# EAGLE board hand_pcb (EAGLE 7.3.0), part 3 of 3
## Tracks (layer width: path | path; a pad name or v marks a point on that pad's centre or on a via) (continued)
N$80 (continued)
  Top 0.381: C64.1 102.23,75.46 102.23,77.09 104.59,79.45 THMB3.9
N$81
  Top 0.381: THMB3.12 107.83,77.36 108.33,76.86 108.33,75.6 C65.1
N$82
  Top 0.381: PKYRNG3.12 105.34,109.19 106.53,110.85 106.81,111.06 107.37,111.91 108.84,111.91 C62.1
N$83
  Top 0.381: C59.1 138.01,108.27 INDMID3.12
N$84
  Top 0.254: O3.3 90.39,81.51 | 92.99,84.48 93.06,84.47 HAND_MICRO3.33
  Top 0.508: 90.39,81.51 91.54,81.51 92.99,82.92 92.99,84.48
N$85
  Top 0.254: O3.1 88.88,83.64 | 91.47,86.31 HAND_MICRO3.32
  Top 0.508: 88.88,83.64 88.88,84.25 90.96,86.31 91.47,86.31
N$86
  Top 0.254: RST3.P$1 85.18,96.05 BOOTLOADER3.10
N$87
  Top 0.254: R51.2 96.36,98.58 95.12,98.58 94.61,98.06 HAND_MICRO3.13
N$88  (via drill 0.38)
  Top 0.254: 94.28,100.87 C68.1 95.43,100.94 95.43,102.31 96.04,102.92 96.72,102.92 97.36,102.28 R51.1 | 94.28,100.87 C67.1 | 94.28,100.87 94.28,98.81 94.11,98.63 HAND_MICRO3.14 94.11,94.92 v93.93,94.59
  Bottom 0.254: v93.93,94.59 94,93.52 U$39.2
N$89  (via drill 0.38)
  Top 0.254: HAND_MICRO3.17 89.62,93.97 v89.59,94 | v91.57,97.89 91.24,97.89 90.47,98.65 90.47,100.38 90.97,100.87 C69.1
  Bottom 0.254: v89.59,94 89.59,95.91 v91.57,97.89
N$90  (via drill 0.38)
  Top 0.254: USB3.4 83.06,105.66 84.23,105.69 84.81,105.11 v84.81,100.53 | v92.59,91.25 92.39,91.25 92.13,90.98 HAND_MICRO3.23 | BOOTLOADER3.6 87.16,90.35 88.19,90.35 v88.72,89.43
  Bottom 0.254: v84.81,100.53 84.81,97.41 90.99,91.25 v92.59,91.25 91.25,89.45 v88.72,89.43
N$91  (via drill 0.38)
  Top 0.254: v109.47,93.45 110.84,93.45 RED3.2
  Bottom 0.254: R62.1 109,92.98 v109.47,93.45
N$92  (via drill 0.38)
  Top 0.254: GREEN3.2 108.96,95.67 v109.98,96.62
  Bottom 0.254: v109.98,96.62 109.79,96.65 R63.1
N$93  (via drill 0.38)
  Top 0.254: v112.62,96.72 111.4,95.83 YELLOW3.2
  Bottom 0.254: R64.1 112.39,96.53 v112.62,96.72
N$94
  Top 0.254: INDMID3.6 128.86,112.05 IMF3.P$1
N$95
  Top 0.254: PKYRNG3.6 102.03,104.73 100.84,103.53 PYF3.P$1
N$96
  Top 0.254: THMB3.6 103.33,82.05 TF3.P$1
OSC
  pour Route15 (isolate 0.406, rank 6): 12.79,13.22 16,13.22 16,13.97 16.9,13.97 18.52,15.58 18.52,17.86 16.87,19.51 15.28,19.51 13.07,17.3 12.79,17.3
  pour Bottom (isolate 0.406, rank 6): 12.79,13.22 16,13.22 16,13.97 16.9,13.97 18.52,15.58 18.52,17.86 16.87,19.51 15.28,19.51 13.07,17.3 12.79,17.3
  pour Route2 (isolate 0.406, rank 6): 12.79,13.22 16,13.22 16,13.97 16.9,13.97 18.52,15.58 18.52,17.86 16.87,19.51 15.28,19.51 13.07,17.3 12.79,17.3
OSC1
  pour Route15 (isolate 0.406, rank 6): 58.97,120.41 55.75,120.41 55.75,119.66 54.85,119.66 53.24,118.05 53.24,115.77 54.89,114.12 56.48,114.12 58.69,116.33 58.97,116.33
  pour Bottom (isolate 0.406, rank 6): 58.97,120.41 55.75,120.41 55.75,119.66 54.85,119.66 53.24,118.05 53.24,115.77 54.89,114.12 56.48,114.12 58.69,116.33 58.97,116.33
  pour Route2 (isolate 0.406, rank 6): 58.97,120.41 55.75,120.41 55.75,119.66 54.85,119.66 53.24,118.05 53.24,115.77 54.89,114.12 56.48,114.12 58.69,116.33 58.97,116.33
OSC2
  pour Route15 (isolate 0.406, rank 6): 133.82,53.25 130.61,53.25 130.61,52.5 129.71,52.5 128.09,50.89 128.09,48.62 129.74,46.96 131.33,46.96 133.54,49.17 133.82,49.17
  pour Bottom (isolate 0.406, rank 6): 133.82,53.25 130.61,53.25 130.61,52.5 129.71,52.5 128.09,50.89 128.09,48.62 129.74,46.96 131.33,46.96 133.54,49.17 133.82,49.17
  pour Route2 (isolate 0.406, rank 6): 133.82,53.25 130.61,53.25 130.61,52.5 129.71,52.5 128.09,50.89 128.09,48.62 129.74,46.96 131.33,46.96 133.54,49.17 133.82,49.17
OSC3
  pour Route15 (isolate 0.406, rank 6): 87.77,80.23 90.98,80.23 90.98,80.98 91.88,80.98 93.5,82.59 93.5,84.86 91.85,86.51 90.26,86.51 88.05,84.3 87.77,84.3
  pour Bottom (isolate 0.406, rank 6): 87.77,80.23 90.98,80.23 90.98,80.98 91.88,80.98 93.5,82.59 93.5,84.86 91.85,86.51 90.26,86.51 88.05,84.3 87.77,84.3
  pour Route2 (isolate 0.406, rank 6): 87.77,80.23 90.98,80.23 90.98,80.98 91.88,80.98 93.5,82.59 93.5,84.86 91.85,86.51 90.26,86.51 88.05,84.3 87.77,84.3
PKY1
  Top 0.254: PKYRNG.5
  Top 0.381: PKYRNG.5 25.55,38.89
  Top 0.635: 25.55,38.89 23.32,38 19.68,41.71 18.37,42.93 PINKY.2
PKY2
  Top 0.381: 22.96,41.25 23.5,40.89 PKYRNG.3
  Top 0.635: 22.96,41.25 19.49,43.54 PINKY.1
PKY3
  Top 0.254: 45.36,94.69 PKYRNG1.5
  Top 0.381: 45.36,94.69 46.2,94.74
  Top 0.635: 46.2,94.74 48.44,95.63 52.07,91.92 53.38,90.7 PINKY1.2
PKY4
  Top 0.381: 48.79,92.38 48.26,92.74 PKYRNG1.3
  Top 0.635: 48.79,92.38 52.26,90.09 PINKY1.1
PKY5
  Top 0.254: PKYRNG2.5
  Top 0.381: PKYRNG2.5 121.06,27.58
  Top 0.635: 121.06,27.58 123.29,28.47 126.92,24.77 128.24,23.55 PINKY2.2
PKY6
  Top 0.381: 123.65,25.22 123.11,25.58 PKYRNG2.3
  Top 0.635: 123.65,25.22 127.11,22.94 PINKY2.1
PKY7
  Top 0.254: PKYRNG3.5
  Top 0.381: PKYRNG3.5 100.53,105.89
  Top 0.635: 100.53,105.89 98.3,105 94.67,108.71 93.35,109.93 PINKY3.2
PKY8
  Top 0.381: 97.94,108.25 98.48,107.9 PKYRNG3.3
  Top 0.635: 97.94,108.25 94.47,110.54 PINKY3.1
PKYENC1  (via drill 0.38)
  Top 0.254: HAND_MICRO.26 16.85,22.47 17.25,22.68 17.32,23.34 v18.24,23.44 | PINKY.5 14.7,42.2 v14.73,42.16
  Route2 0.254: v14.73,42.16 14.73,28.32 18.34,24.71 18.34,23.55 v18.24,23.44
PKYENC2  (via drill 0.38, 0.39)
  Top 0.254: HAND_MICRO.27 17.01,21.97 17.02,21.97 17.3,21.97 18.01,22.63 18.62,22.63 v19.05,22.89 | v15.9,40.13 PINKY.4
  Route2 0.254: v19.05,22.89 19.13,25.02 15.65,28.5 15.65,36.12 17.07,37.54 17.07,38.96 v15.9,40.13
PKYENC3  (via drill 0.38)
  Top 0.254: HAND_MICRO1.26 54.9,111.16 54.51,110.95 54.43,110.29 v53.52,110.19 | PINKY1.5 57.05,91.43 v57.02,91.47
  Route2 0.254: v57.02,91.47 57.02,105.31 53.42,108.92 53.42,110.08 v53.52,110.19
PKYENC4  (via drill 0.38, 0.39)
  Top 0.254: HAND_MICRO1.27 54.74,111.66 54.46,111.66 53.75,111 53.14,111 v52.7,110.74 | v55.85,93.5 PINKY1.4
  Route2 0.254: v52.7,110.74 52.63,108.61 56.11,105.13 56.11,97.51 54.69,96.09 54.69,94.67 v55.85,93.5
PKYENC5  (via drill 0.38)
  Top 0.254: HAND_MICRO2.26 129.76,44.01 129.36,43.79 129.29,43.13 v128.37,43.03 | PINKY2.5 131.91,24.28 v131.88,24.31
  Route2 0.254: v131.88,24.31 131.88,38.15 128.27,41.76 128.27,42.93 v128.37,43.03
PKYENC6  (via drill 0.38, 0.39)
  Top 0.254: HAND_MICRO2.27 129.59,44.51 129.59,44.5 129.31,44.5 128.6,43.84 127.99,43.84 v127.56,43.59 | v130.71,26.34 PINKY2.4
  Route2 0.254: v127.56,43.59 127.48,41.45 130.96,37.97 130.96,30.35 129.54,28.93 129.54,27.51 v130.71,26.34
PKYENC7  (via drill 0.38)
  Top 0.254: HAND_MICRO3.26 91.83,89.47 92.23,89.69 92.3,90.35 v93.22,90.45 | PINKY3.5 89.68,109.2 v89.71,109.17
  Route2 0.254: v89.71,109.17 89.71,95.33 93.32,91.72 93.32,90.55 v93.22,90.45
PKYENC8  (via drill 0.38, 0.39)
  Top 0.254: HAND_MICRO3.27 91.99,88.97 92,88.98 92.28,88.98 92.99,89.64 93.6,89.64 v94.03,89.89 | v90.88,107.14 PINKY3.4
  Route2 0.254: v94.03,89.89 94.11,92.02 90.63,95.5 90.63,103.12 92.05,104.55 92.05,105.97 v90.88,107.14
PKYISEN  (via drill 0.38)
  Top 0.254: HAND_MICRO.9 21.63,30.32 v22.2,30.89
  Top 0.381: PKYRNG.4 25.07,40.03
  Top 0.635: 25.07,40.03 v23.39,39.78
  Bottom 0.254: v22.2,30.89 23.39,32.08 v23.39,39.78
  Bottom 0.635: v23.39,39.78 25.45,38.18 R9.2
PKYISEN1  (via drill 0.38)
  Top 0.254: HAND_MICRO1.9 50.13,103.31 v49.55,102.74
  Top 0.381: PKYRNG1.4 46.69,93.6
  Top 0.635: 46.69,93.6 v48.36,93.85
  Bottom 0.254: v49.55,102.74 48.36,101.55 v48.36,93.85
  Bottom 0.635: v48.36,93.85 46.3,95.45 R25.2
PKYISEN2  (via drill 0.38)
  Top 0.254: HAND_MICRO2.9 124.98,36.16 v124.41,35.59
  Top 0.381: PKYRNG2.4 121.54,26.44
  Top 0.635: 121.54,26.44 v123.22,26.7
  Bottom 0.254: v124.41,35.59 123.22,34.39 v123.22,26.7
  Bottom 0.635: v123.22,26.7 121.16,28.3 R41.2
PKYISEN3  (via drill 0.38)
  Top 0.254: HAND_MICRO3.9 96.61,97.32 v97.18,97.89
  Top 0.381: PKYRNG3.4 100.05,107.04
  Top 0.635: 100.05,107.04 v98.37,106.78
  Bottom 0.254: v97.18,97.89 98.37,99.08 v98.37,106.78
  Bottom 0.635: v98.37,106.78 100.43,105.18 R57.2
PKYPWM1
  Top 0.254: 27.69,38.92 PKYRNG.7 27.71,37.54 27.48,37.31 27.48,29.13 22.91,24.56 22.05,24.56 19.63,22.15 18.26,22.15 17.58,21.47 HAND_MICRO.28
PKYPWM2
  Top 0.254: 28.37,38.92 PKYRNG.8 28.35,37.24 27.99,36.88 27.99,28.88 23.22,24.11 22.33,24.11 19.84,21.61 18.47,21.61 17.82,20.97 HAND_MICRO.29
PKYPWM3
  Top 0.254: 43.38,94.71 PKYRNG1.8 43.4,96.39 43.76,96.75 43.76,104.75 48.54,109.53 49.43,109.53 51.92,112.01 53.29,112.01 53.94,112.66 HAND_MICRO1.29
PKYPWM4
  Top 0.254: 44.07,94.7 PKYRNG1.7 44.04,96.09 44.27,96.32 44.27,104.5 48.84,109.07 49.71,109.07 52.12,111.48 53.49,111.48 54.17,112.16 HAND_MICRO1.28
PKYPWM5
  Top 0.254: 118.24,27.55 PKYRNG2.8 118.26,29.23 118.62,29.59 118.62,37.59 123.39,42.37 124.28,42.37 126.77,44.86 128.14,44.86 128.79,45.51 HAND_MICRO2.29
PKYPWM6
  Top 0.254: 118.92,27.55 PKYRNG2.7 118.9,27.54 118.9,28.93 119.13,29.16 119.13,37.34 123.7,41.91 124.56,41.91 126.97,44.32 128.35,44.32 129.03,45.01 HAND_MICRO2.28
PKYPWM7
  Top 0.254: 103.35,105.93 PKYRNG3.8 103.33,104.25 102.97,103.89 102.97,95.89 98.2,91.11 97.31,91.11 94.82,88.62 93.45,88.62 92.8,87.97 HAND_MICRO3.29
PKYPWM8
  Top 0.254: 102.67,105.93 PKYRNG3.7 102.69,105.94 102.69,104.55 102.46,104.32 102.46,96.14 97.89,91.57 97.03,91.57 94.61,89.15 93.24,89.15 92.56,88.47 HAND_MICRO3.28
RNG1
  Top 0.254: PKYRNG.16
  Top 0.381: PKYRNG.16 26.39,44.91
  Top 0.635: 26.39,44.91 26.39,46.28 31.34,46.28 32.49,47.37 32.49,47.73 32.49,48.34 RING.1
RNG2
  Top 0.381: 23.39,42.32 23.95,41.54 PKYRNG.2
  Top 0.635: 23.39,42.32 22.5,43.89 24.89,47.37 30.76,47.37 31.27,48.11 31.27,49.33 31.3,49.33 RING.2
RNG3
  Top 0.254: 45.36,90.14 PKYRNG1.16
  Top 0.381: 45.36,90.14 45.36,88.72
  Top 0.635: 45.36,88.72 45.36,87.35 40.41,87.35 39.27,86.26 39.27,85.9 39.26,85.29 RING1.1
RNG4
  Top 0.381: 48.36,91.31 47.8,92.09 PKYRNG1.2
  Top 0.635: 48.36,91.31 49.25,89.74 46.86,86.26 41,86.26 40.49,85.52 40.49,84.3 40.46,84.3 RING1.2
RNG5
  Top 0.254: PKYRNG2.16
  Top 0.381: PKYRNG2.16 120.22,21.57
  Top 0.635: 120.22,21.57 120.22,20.19 115.27,20.19 114.12,19.1 114.12,18.75 114.11,18.14 RING2.1
RNG6
  Top 0.381: 123.22,24.16 122.66,24.93 PKYRNG2.2
  Top 0.635: 123.22,24.16 124.1,22.58 121.72,19.1 115.85,19.1 115.34,18.36 115.34,17.14 115.31,17.14 RING2.2
RNG7
  Top 0.254: PKYRNG3.16
  Top 0.381: PKYRNG3.16 101.37,111.91
  Top 0.635: 101.37,111.91 101.37,113.28 106.32,113.28 107.47,114.38 107.47,114.73 107.47,115.34 RING3.1
RNG8
  Top 0.381: 98.37,109.32 98.93,108.55 PKYRNG3.2
  Top 0.635: 98.37,109.32 97.48,110.9 99.87,114.38 105.74,114.38 106.25,115.11 106.25,116.33 106.28,116.33 RING3.2
RNGENC1  (via drill 0.38)
  Top 0.254: HAND_MICRO.2 25.13,27.85 v24.38,27.48 | v27.15,48.72 27.71,49.66 RING.5
  Route2 0.254: v24.38,27.48 24.77,28.98 25.91,30.12 25.91,33.48 21.69,37.69 21.69,45.59 24.46,48.56 26.85,48.69 v27.15,48.72
RNGENC2  (via drill 0.38)
  Top 0.254: RING.4 28.85,49.14 v28.68,48.64 | v26.7,31.01 25.64,29.97 HAND_MICRO.1
  Route2 0.254: v28.68,48.64 28.04,47.95 24.87,47.73 22.55,45.14 22.55,38.15 27,33.71 27,31.32 v26.7,31.01
RNGENC3  (via drill 0.38)
  Top 0.254: RING1.4 42.91,84.49 v43.08,84.99 | v45.06,102.62 46.11,103.66 HAND_MICRO1.1
  Route2 0.254: v43.08,84.99 43.71,85.67 46.89,85.9 49.2,88.49 49.2,95.48 44.76,99.92 44.76,102.31 v45.06,102.62
RNGENC4  (via drill 0.38)
  Top 0.254: HAND_MICRO1.2 46.63,105.78 v47.37,106.15 | v44.6,84.91 44.04,83.97 RING1.5
  Route2 0.254: v47.37,106.15 46.99,104.65 45.85,103.5 45.85,100.15 50.06,95.94 50.06,88.04 47.3,85.06 44.91,84.94 v44.6,84.91
RNGENC5  (via drill 0.38)
  Top 0.254: RING2.4 117.76,17.33 v117.93,17.83 | v119.91,35.46 120.97,36.5 HAND_MICRO2.1
  Route2 0.254: v117.93,17.83 118.57,18.52 121.74,18.75 124.05,21.34 124.05,28.32 119.61,32.77 119.61,35.15 v119.91,35.46
RNGENC6  (via drill 0.38)
  Top 0.254: HAND_MICRO2.2 121.48,38.63 v122.22,38.99 | v119.46,17.75 118.9,16.81 RING2.5
  Route2 0.254: v122.22,38.99 121.84,37.49 120.7,36.35 120.7,32.99 124.92,28.78 124.92,20.88 122.15,17.91 119.76,17.78 v119.46,17.75
RNGENC7  (via drill 0.38)
  Top 0.254: RING3.4 103.83,116.15 v103.66,115.65 | v101.68,98.02 100.62,96.98 HAND_MICRO3.1
  Route2 0.254: v103.66,115.65 103.02,114.96 99.85,114.73 97.54,112.14 97.54,105.16 101.98,100.71 101.98,98.32 v101.68,98.02
RNGENC8  (via drill 0.38)
  Top 0.254: HAND_MICRO3.2 100.11,94.85 v99.36,94.49 | v102.13,115.72 102.69,116.66 RING3.5
  Route2 0.254: v99.36,94.49 99.75,95.99 100.89,97.13 100.89,100.48 96.67,104.7 96.67,112.6 99.44,115.57 101.83,115.7 v102.13,115.72
RNGISEN  (via drill 0.38)
  Top 0.254: HAND_MICRO.10 21.13,29.95 v20.62,30.45
  Top 0.381: PKYRNG.1 24.71,42.35
  Top 0.635: 24.71,42.35 v23.98,43.84
  Bottom 0.254: v20.62,30.45 22.17,32 22.17,41.43 23.98,43.23 v23.98,43.84
  Bottom 0.635: v23.98,43.84 24.38,44.25 R8.2
RNGISEN1  (via drill 0.38)
  Top 0.254: HAND_MICRO1.10 50.63,103.68 v51.13,103.17
  Top 0.381: PKYRNG1.1 47.04,91.28
  Top 0.635: 47.04,91.28 v47.78,89.79
  Bottom 0.254: v51.13,103.17 49.58,101.62 49.58,92.2 47.78,90.4 v47.78,89.79
  Bottom 0.635: v47.78,89.79 47.37,89.38 R24.2
RNGISEN2  (via drill 0.38)
  Top 0.254: HAND_MICRO2.10 125.48,36.52 v125.98,36.02
  Top 0.381: PKYRNG2.1 121.89,24.12
  Top 0.635: 121.89,24.12 v122.63,22.63
  Bottom 0.254: v125.98,36.02 124.44,34.47 124.44,25.04 122.63,23.24 v122.63,22.63
  Bottom 0.635: v122.63,22.63 122.22,22.23 R40.2
RNGISEN3  (via drill 0.38)
  Top 0.254: HAND_MICRO3.10 96.11,96.96 v95.61,97.46
  Top 0.381: PKYRNG3.1 99.69,109.36
  Top 0.635: 99.69,109.36 v98.96,110.85
  Bottom 0.254: v95.61,97.46 97.16,99.01 97.16,108.43 98.96,110.24 v98.96,110.85
  Bottom 0.635: v98.96,110.85 99.36,111.25 R56.2
RNGPWM1  (via drill 0.38)
  Top 0.254: PKYRNG.14 27.7,44.65 27.99,44.93 v30.26,44.79 | HAND_MICRO.46 24.63,18.55 24.4,18.78 23.25,18.78 v23.02,19.01
  Route2 0.254: v23.02,19.01 23.02,24.98 27.85,29.81 27.85,37.92 30.26,40.34 v30.26,44.79
RNGPWM2  (via drill 0.38)
  Top 0.254: PKYRNG.13 30.05,43.49 v31.32,44.83 | HAND_MICRO.49 v26.62,18.67
  Route2 0.254: v31.32,44.83 31.32,43.8 30.85,43.33 30.85,40.21 28.28,37.64 28.28,29.65 23.43,24.8 23.43,20.77 24.82,18.69 v26.62,18.67
RNGPWM3  (via drill 0.38)
  Top 0.254: PKYRNG1.13 41.7,90.14 v40.44,88.8 | HAND_MICRO1.49 v45.14,114.96
  Route2 0.254: v40.44,88.8 40.44,89.83 40.91,90.3 40.91,93.42 43.47,95.99 43.47,103.97 48.32,108.83 48.32,112.86 46.94,114.94 v45.14,114.96
RNGPWM4  (via drill 0.38)
  Top 0.254: PKYRNG1.14 44.05,88.98 43.76,88.7 v41.49,88.84 | HAND_MICRO1.46 47.13,115.08 47.36,114.85 48.5,114.85 v48.73,114.62
  Route2 0.254: v48.73,114.62 48.73,108.65 43.9,103.82 43.9,95.71 41.49,93.29 v41.49,88.84
RNGPWM5  (via drill 0.38)
  Top 0.254: PKYRNG2.13 116.55,22.98 v115.29,21.64 | HAND_MICRO2.49 v119.99,47.8
  Route2 0.254: v115.29,21.64 115.29,22.67 115.76,23.14 115.76,26.26 118.33,28.83 118.33,36.82 123.18,41.67 123.18,45.71 121.79,47.78 v119.99,47.8
RNGPWM6  (via drill 0.38)
  Top 0.254: PKYRNG2.14 118.91,21.83 118.62,21.54 v116.34,21.68 | HAND_MICRO2.46 121.98,47.92 122.21,47.69 123.36,47.69 v123.58,47.46
  Route2 0.254: v123.58,47.46 123.58,41.49 118.76,36.66 118.76,28.55 116.34,26.14 v116.34,21.68
RNGPWM7  (via drill 0.38)
  Top 0.254: PKYRNG3.13 105.04,110.5 v106.3,111.84 | HAND_MICRO3.49 v101.6,85.67
  Route2 0.254: v106.3,111.84 106.3,110.81 105.83,110.34 105.83,107.21 103.26,104.65 103.26,96.66 98.41,91.81 98.41,87.77 99.8,85.7 v101.6,85.67
RNGPWM8  (via drill 0.38)
  Top 0.254: PKYRNG3.14 102.68,111.65 102.97,111.94 v105.25,111.8 | HAND_MICRO3.46 99.61,85.56 99.38,85.79 98.23,85.79 v98.01,86.02
  Route2 0.254: v98.01,86.02 98.01,91.99 102.83,96.81 102.83,104.93 105.25,107.34 v105.25,111.8
SCL0  (via drill 0.38, 0.39)
  Top 0.254: v20.45,18.9 20.13,18.73 HAND_MICRO.37 20.13,15.53 20.65,15.01 20.65,12.62 R10.1 18.53,13.42 v17.27,13.21 | U$1.14 47.16,44.12 48.36,42.93 50.09,42.93 U$7.C
  Route2 0.254: U$8.C 65.48,50.75 63.27,50.75 59.64,52.73 58.14,53.98 53.65,53.98 52.73,53.06 43.43,53.06 43.1,53.39 42.53,53.5 | 42.53,53.5 39.04,54.15 U$5.C 37.21,53.24 33.27,53.24 31.32,51.28 31.32,47.4 34.14,44.58 34.14,42.8 32.26,40.92 32.26,32.13 26.01,25.88 v26.11,25.48 | U$7.C 50.01,44.88 48.59,44.88 45.74,47.73 44.55,47.73 44.02,48.26 43.71,48.26 42.65,49.33 42.65,53.38 42.53,53.5 | v17.27,13.21 17.27,11.63 18.54,10.44 U$11.SCL
  Route15 0.254: v20.45,18.9 20.95,19.56 21.41,19.79 24.18,24.69 v26.11,25.48
SCL1  (via drill 0.38, 0.39)
  Top 0.254: HAND_MICRO.55 26.66,22.47 25.6,20.7 v25.65,20.34
  Route2 0.254: U$12.SCL 7.29,17.25 11.25,17.25 13.82,19.74 19.38,19.74 v19.61,19.51
  Bottom 0.254: R12.1 23.23,20.83 | 23.23,20.83 v25.65,20.34 | v19.61,19.51 20.02,19.91 20.19,19.91 21.34,20.24 23.23,20.83
SCL2  (via drill 0.38, 0.39)
  Top 0.254: v51.31,114.73 51.63,114.9 HAND_MICRO1.37 51.63,118.1 51.1,118.62 51.1,121.01 R26.1 53.23,120.21 v54.48,120.42 | U$13.14 24.59,89.51 23.39,90.7 21.67,90.7 U$18.C
  Route2 0.254: U$20.C 6.27,82.88 8.48,82.88 12.12,80.9 13.61,79.65 18.11,79.65 19.02,80.57 28.32,80.57 28.65,80.24 29.22,80.13 | 29.22,80.13 32.72,79.48 U$17.C 34.54,80.39 38.48,80.39 40.44,82.35 40.44,86.23 37.62,89.05 37.62,90.83 39.5,92.71 39.5,101.5 45.74,107.75 v45.64,108.15 | U$18.C 21.74,88.75 23.16,88.75 26.01,85.9 27.2,85.9 27.74,85.37 28.04,85.37 29.11,84.3 29.11,80.25 29.22,80.13 | v54.48,120.42 54.48,122 53.21,123.19 U$23.SCL
  Route15 0.254: v51.31,114.73 50.8,114.07 50.34,113.84 47.57,108.94 v45.64,108.15
SCL3  (via drill 0.38, 0.39)
  Top 0.254: HAND_MICRO1.55 45.1,111.16 46.15,112.93 v46.1,113.28
  Route2 0.254: U$24.SCL 64.47,116.38 60.5,116.38 57.94,113.89 52.38,113.89 v52.15,114.12
  Bottom 0.254: R28.1 48.53,112.8 | 48.53,112.8 v46.1,113.28 | v52.15,114.12 51.74,113.72 51.56,113.72 50.42,113.39 48.53,112.8
SCL4  (via drill 0.38, 0.39)
  Top 0.254: v126.16,47.57 126.48,47.74 HAND_MICRO2.37 126.48,50.94 125.96,51.46 125.96,53.85 R42.1 128.08,53.05 v129.34,53.26 | U$25.14 99.44,22.35 98.25,23.55 96.52,23.55 U$30.C
  Route2 0.254: U$32.C 81.13,15.72 83.34,15.72 86.97,13.74 88.47,12.5 92.96,12.5 93.88,13.41 103.17,13.41 103.5,13.08 104.08,12.97 | 104.08,12.97 107.57,12.32 U$29.C 109.4,13.23 113.33,13.23 115.29,15.19 115.29,19.07 112.47,21.89 112.47,23.67 114.35,25.55 114.35,34.34 120.6,40.59 v120.5,41 | U$30.C 96.6,21.59 98.02,21.59 100.86,18.75 102.06,18.75 102.59,18.21 102.89,18.21 103.96,17.14 103.96,13.09 104.08,12.97 | v129.34,53.26 129.34,54.84 128.07,56.03 U$35.SCL
  Route15 0.254: v126.16,47.57 125.65,46.91 125.2,46.69 122.43,41.78 v120.5,41
SCL5  (via drill 0.38, 0.39)
  Top 0.254: HAND_MICRO2.55 119.95,44.01 121.01,45.77 v120.95,46.13
  Route2 0.254: U$36.SCL 139.32,49.23 135.36,49.23 132.79,46.74 127.23,46.74 v127,46.97
  Bottom 0.254: R44.1 123.38,45.64 | 123.38,45.64 v120.95,46.13 | v127,46.97 126.59,46.56 126.42,46.56 125.27,46.23 123.38,45.64
SCL6  (via drill 0.38, 0.39)
  Top 0.254: v95.43,85.9 95.11,85.74 HAND_MICRO3.37 95.11,82.54 95.63,82.02 95.63,79.63 R58.1 93.51,80.43 v92.25,80.21 | U$37.14 122.15,111.13 123.34,109.93 125.07,109.93 U$42.C
  Route2 0.254: U$44.C 140.46,117.75 138.25,117.75 134.62,119.74 133.12,120.98 128.63,120.98 127.71,120.07 118.42,120.07 118.08,120.4 117.51,120.5 | 117.51,120.5 114.02,121.16 U$41.C 112.19,120.24 108.25,120.24 106.3,118.29 106.3,114.4 109.12,111.58 109.12,109.8 107.24,107.92 107.24,99.14 100.99,92.89 v101.09,92.48 | U$42.C 124.99,111.89 123.57,111.89 120.73,114.73 119.53,114.73 119,115.27 118.69,115.27 117.63,116.33 117.63,120.39 117.51,120.5 | v92.25,80.21 92.25,78.64 93.52,77.44 U$47.SCL
  Route15 0.254: v95.43,85.9 95.94,86.56 96.39,86.79 99.16,91.69 v101.09,92.48
SCL7  (via drill 0.38, 0.39)
  Top 0.254: HAND_MICRO3.55 101.64,89.47 100.58,87.71 v100.64,87.35
  Route2 0.254: U$48.SCL 82.27,84.25 86.23,84.25 88.8,86.74 94.36,86.74 v94.59,86.51
  Bottom 0.254: R60.1 98.21,87.83 | 98.21,87.83 v100.64,87.35 | v94.59,86.51 95,86.92 95.17,86.92 96.32,87.25 98.21,87.83
SDA0  (via drill 0.38, 0.39)
  Top 0.254: HAND_MICRO.38 20.63,16.05 21.23,15.44 | 21.23,15.44 21.23,13.12 R11.1 | U$1.15 48.22,44.77 U$7.D | v39.37,52.98 39.14,53.21 37.16,53.21 U$5.D | v21.39,16.05 21.23,15.9 21.23,15.44
  Route2 0.254: U$8.D 62.99,52.7 53.34,57.33 49.17,57.25 43.75,56.08 39.32,55.12 37.19,55.12 U$5.D 32.87,54.15 30.86,52.15 30.86,47.09 33.68,44.27 33.68,43.08 31.8,41.2 31.8,32.41 24.89,25.5 v25.09,23.8 | U$7.D 48.84,43.87 45.44,47.27 43.94,47.27 42.14,49.07 42.14,50.22 v39.37,52.98 | U$11.SDA 19.41,8.38 19.41,11.18 18.31,12.27 v18.31,12.62
  Route15 0.254: v25.09,23.8 23.44,21.84 23.14,20.22 21.39,18.47 v21.39,16.05
  Bottom 0.254: v18.31,12.62 18.95,13.36 21.23,13.36 21.39,13.51 v21.39,16.05
SDA1  (via drill 0.38, 0.39)
  Top 0.254: HAND_MICRO.56 26.37,22.97 25.66,21.77 25.38,21.41 v24.54,21.54 20.98,21.54 v20.47,21.03
  Route2 0.254: U$12.SDA 6.96,20.37 9.65,20.37 10.72,19.3 12.14,19.3 13.74,20.9 18.8,21.34 v20.47,21.03
  Bottom 0.254: v24.54,21.54 24.46,21.97 24.36,22.84 23.75,23.14 R13.1
SDA2  (via drill 0.38, 0.39)
  Top 0.254: HAND_MICRO1.38 51.13,117.58 50.52,118.19 | 50.52,118.19 50.52,120.51 R27.1 | U$13.15 23.54,88.86 U$18.D | v32.38,80.64 32.61,80.42 34.59,80.42 U$17.D | v50.37,117.58 50.52,117.73 50.52,118.19
  Route2 0.254: U$20.D 8.76,80.92 18.41,76.3 22.58,76.38 28.01,77.55 32.44,78.51 34.57,78.51 U$17.D 38.89,79.48 40.89,81.48 40.89,86.54 38.08,89.36 38.08,90.55 39.95,92.43 39.95,101.22 46.86,108.13 v46.66,109.83 | U$18.D 22.91,89.76 26.31,86.36 27.81,86.36 29.62,84.56 29.62,83.41 v32.38,80.64 | U$23.SDA 52.35,125.25 52.35,122.45 53.44,121.36 v53.44,121.01
  Route15 0.254: v46.66,109.83 48.31,111.78 48.62,113.41 50.37,115.16 v50.37,117.58
  Bottom 0.254: v53.44,121.01 52.81,120.27 50.52,120.27 50.37,120.12 v50.37,117.58
SDA3  (via drill 0.38, 0.39)
  Top 0.254: HAND_MICRO1.56 45.38,110.66 46.1,111.86 46.38,112.22 v47.22,112.09 50.77,112.09 v51.28,112.6
  Route2 0.254: U$24.SDA 64.8,113.26 62.1,113.26 61.04,114.33 59.61,114.33 58.01,112.72 52.96,112.29 v51.28,112.6
  Bottom 0.254: v47.22,112.09 47.3,111.66 47.4,110.8 48.01,110.49 R29.1
SDA4  (via drill 0.38, 0.39)
  Top 0.254: HAND_MICRO2.38 125.98,50.42 125.37,51.03 | 125.37,51.03 125.37,53.35 R43.1 | U$25.15 98.39,21.7 U$30.D | v107.24,13.49 107.47,13.26 109.45,13.26 U$29.D | v125.22,50.42 125.37,50.57 125.37,51.03
  Route2 0.254: U$32.D 83.62,13.77 93.27,9.14 97.43,9.22 102.86,10.39 107.29,11.35 109.42,11.35 U$29.D 113.74,12.32 115.75,14.33 115.75,19.38 112.93,22.2 112.93,23.39 114.81,25.27 114.81,34.06 121.72,40.97 v121.51,42.67 | U$30.D 97.77,22.61 101.17,19.2 102.67,19.2 104.47,17.4 104.47,16.26 v107.24,13.49 | U$35.SDA 127.2,58.09 127.2,55.3 128.29,54.2 v128.29,53.85
  Route15 0.254: v121.51,42.67 123.17,44.63 123.47,46.25 125.22,48.01 v125.22,50.42
  Bottom 0.254: v128.29,53.85 127.66,53.11 125.37,53.11 125.22,52.96 v125.22,50.42
SDA5  (via drill 0.38, 0.39)
  Top 0.254: HAND_MICRO2.56 120.24,43.51 120.95,44.7 121.23,45.06 v122.07,44.93 125.63,44.93 v126.14,45.44
  Route2 0.254: U$36.SDA 139.65,46.1 136.96,46.1 135.89,47.17 134.47,47.17 132.87,45.57 127.81,45.14 v126.14,45.44
  Bottom 0.254: v122.07,44.93 122.15,44.5 122.25,43.64 122.86,43.33 R45.1
SDA6  (via drill 0.38, 0.39)
  Top 0.254: HAND_MICRO3.38 95.61,83.06 96.22,82.45 | 96.22,82.45 96.22,80.12 R59.1 | U$37.15 123.2,111.78 U$42.D | v114.35,119.99 114.12,120.22 112.14,120.22 U$41.D | v96.37,83.06 96.22,82.91 96.22,82.45
  Route2 0.254: U$44.D 137.97,119.71 128.32,124.33 124.16,124.26 118.73,123.08 114.3,122.12 112.17,122.12 U$41.D 107.85,121.16 105.84,119.15 105.84,114.1 108.66,111.28 108.66,110.08 106.78,108.2 106.78,99.42 99.87,92.51 v100.08,90.81 | U$42.D 123.83,110.87 120.42,114.28 118.92,114.28 117.12,116.08 117.12,117.22 v114.35,119.99 | U$47.SDA 94.39,75.39 94.39,78.18 93.29,79.27 v93.29,79.63
  Route15 0.254: v100.08,90.81 98.42,88.85 98.12,87.22 96.37,85.47 v96.37,83.06
  Bottom 0.254: v93.29,79.63 93.93,80.37 96.22,80.37 96.37,80.52 v96.37,83.06
SDA7  (via drill 0.38, 0.39)
  Top 0.254: HAND_MICRO3.56 101.35,89.97 100.64,88.78 100.36,88.42 v99.52,88.54 95.96,88.54 v95.45,88.04
  Route2 0.254: U$48.SDA 81.94,87.38 84.63,87.38 85.7,86.31 87.12,86.31 88.72,87.91 93.78,88.34 v95.45,88.04
  Bottom 0.254: v99.52,88.54 99.44,88.98 99.34,89.84 98.73,90.14 R61.1
THA1
  Top 0.381: 35.84,15.72 35.53,15.69 THMB.16
  Top 0.635: 35.84,15.72 36.37,15.34 36.83,14.5 36.83,11.76 37.36,11.23 THUMB_A.1
THA2
  Top 0.381: 32.72,18.62 32.18,18.16 32.2,18.14 THMB.2
  Top 0.635: 32.72,18.62 35.71,19.68 36.91,16.48 37.9,14.81 37.9,12.68 38.12,12.42 THUMB_A.2
THA3
  Top 0.381: 35.92,117.91 36.22,117.94 THMB1.16
  Top 0.635: 35.92,117.91 35.38,118.29 34.92,119.13 34.92,121.87 34.39,122.4 THUMB_A1.1
THA4
  Top 0.381: 39.04,115.01 39.57,115.47 39.55,115.49 THMB1.2
  Top 0.635: 39.04,115.01 36.04,113.94 34.85,117.14 33.86,118.82 33.86,120.95 33.63,121.21 THUMB_A1.2
THA5
  Top 0.381: 110.77,50.75 111.07,50.78 THMB2.16
  Top 0.635: 110.77,50.75 110.24,51.13 109.78,51.97 109.78,54.71 109.25,55.24 106.53,55.24 THUMB_A2.1
THA6
  Top 0.381: 113.89,47.85 114.43,48.31 114.41,48.33 THMB2.2
  Top 0.635: 113.89,47.85 110.9,46.79 109.7,49.99 108.71,51.66 108.71,53.8 108.48,54.05 THUMB_A2.2
THA7
  Top 0.381: 110.82,82.73 110.52,82.7 THMB3.16
  Top 0.635: 110.82,82.73 111.35,82.35 111.81,81.51 111.81,78.77 112.34,78.23 115.06,78.23 THUMB_A3.1
THA8
  Top 0.381: 107.7,85.62 107.16,85.17 107.18,85.14 THMB3.2
  Top 0.635: 107.7,85.62 110.69,86.69 111.89,83.49 112.88,81.81 112.88,79.68 113.11,79.42 THUMB_A3.2
THAENC1  (via drill 0.38)
  Top 0.254: THUMB_A.5 39.91,15.89 39.27,16.74 39.27,17.91 v38.84,18.34 | HAND_MICRO.35 19.13,15.85 18.69,15.42 v18.69,14.43
  Route2 0.254: v38.84,18.34 38.94,18.34 39.4,17.88 39.4,13.36 35.69,9.7 23.72,9.7 v18.69,14.43
THAENC2  (via drill 0.38)
  Top 0.254: THUMB_A.4 39.26,14.82 39.09,14.99 39.09,15.8 v38.41,17.4 | HAND_MICRO.36 19.63,14.84 v19.81,14.66
  Route2 0.254: v38.41,17.4 38.41,13.36 35.23,10.26 24.33,10.26 v19.81,14.66
THAENC3  (via drill 0.38)
  Top 0.254: THUMB_A1.4 32.49,118.81 32.66,118.64 32.66,117.83 v33.35,116.23 | HAND_MICRO1.36 52.13,118.79 v51.94,118.97
  Route2 0.254: v33.35,116.23 33.35,120.27 36.52,123.37 47.42,123.37 v51.94,118.97
THAENC4  (via drill 0.38)
  Top 0.254: THUMB_A1.5 31.84,117.74 32.49,116.89 32.49,115.72 v32.92,115.29 | HAND_MICRO1.35 52.63,117.78 53.06,118.21 v53.06,119.2
  Route2 0.254: v32.92,115.29 32.82,115.29 32.36,115.75 32.36,120.27 36.07,123.93 48.03,123.93 v53.06,119.2
THAENC5  (via drill 0.38)
  Top 0.254: THUMB_A2.4 107.35,51.66 107.52,51.49 107.52,50.67 v108.2,49.07 | HAND_MICRO2.36 126.98,51.63 v126.8,51.82
  Route2 0.254: v108.2,49.07 108.2,53.11 111.38,56.21 122.28,56.21 v126.8,51.82
THAENC6  (via drill 0.38)
  Top 0.254: THUMB_A2.5 106.69,50.58 107.34,49.73 107.34,48.56 v107.77,48.13 | HAND_MICRO2.35 127.48,50.62 127.91,51.05 v127.91,52.05
  Route2 0.254: v107.77,48.13 107.67,48.13 107.21,48.59 107.21,53.11 110.92,56.77 122.89,56.77 v127.91,52.05
THAENC7  (via drill 0.38)
  Top 0.254: THUMB_A3.4 114.24,81.82 114.07,81.99 114.07,82.8 v113.39,84.4 | HAND_MICRO3.36 94.61,81.84 v94.79,81.66
  Route2 0.254: v113.39,84.4 113.39,80.37 110.21,77.27 99.31,77.27 v94.79,81.66
THAENC8  (via drill 0.38)
  Top 0.254: THUMB_A3.5 114.89,82.89 114.25,83.74 114.25,84.91 v113.82,85.34 | HAND_MICRO3.35 94.11,82.86 93.67,82.42 v93.67,81.43
  Route2 0.254: v113.82,85.34 113.92,85.34 114.38,84.89 114.38,80.37 110.67,76.71 98.7,76.71 v93.67,81.43
THAISEN  (via drill 0.38)
  Top 0.254: HAND_MICRO.11 20.63,27.23 v21.01,26.85
  Top 0.381: THMB.1 33.03,17.6
  Top 0.635: 33.03,17.6 v34.95,18.03
  Route2 0.254: v21.01,26.85 21.01,25.6 22.2,24.87 22.25,20.12 22.28,18.58 23.1,17.6 28.42,17.6 29.34,18.52 34.47,18.52 v34.95,18.03
  Bottom 0.635: v34.95,18.03 34.92,18.01 R4.2
THAISEN1  (via drill 0.38)
  Top 0.254: HAND_MICRO1.11 51.13,106.4 v50.75,106.78
  Top 0.381: THMB1.1 38.72,116.03
  Top 0.635: 38.72,116.03 v36.8,115.59
  Route2 0.254: v50.75,106.78 50.75,108.03 49.55,108.76 49.51,113.51 49.48,115.05 48.65,116.03 43.33,116.03 42.42,115.11 37.29,115.11 v36.8,115.59
  Bottom 0.635: v36.8,115.59 36.83,115.62 R20.2
THAISEN2  (via drill 0.38)
  Top 0.254: HAND_MICRO2.11 125.98,39.25 v125.6,39.62
  Top 0.381: THMB2.1 113.58,48.87
  Top 0.635: 113.58,48.87 v111.66,48.44
  Route2 0.254: v125.6,39.62 125.6,40.87 124.41,41.6 124.36,46.35 124.33,47.89 123.51,48.87 118.19,48.87 117.27,47.95 112.14,47.95 v111.66,48.44
  Bottom 0.635: v111.66,48.44 111.68,48.46 R36.2
THAISEN3  (via drill 0.38)
  Top 0.254: HAND_MICRO3.11 95.61,94.23 v95.99,93.85
  Top 0.381: THMB3.1 108.01,84.61
  Top 0.635: 108.01,84.61 v109.93,85.04
  Route2 0.254: v95.99,93.85 95.99,92.61 97.18,91.87 97.23,87.12 97.26,85.58 98.08,84.61 103.4,84.61 104.32,85.52 109.45,85.52 v109.93,85.04
  Bottom 0.635: v109.93,85.04 109.91,85.01 R52.2
THAPWM1  (via drill 0.38)
  Top 0.254: THMB.14 34.19,14.35 35.23,14.35 35.61,13.97 35.61,13.49 35.13,13.01 v35.13,11.6 | v22.12,14.35 v22.13,14.36 HAND_MICRO.41
  Route2 0.254: v35.13,11.6 34.29,10.79 26.82,10.79 23.27,14.35 v22.12,14.35
THAPWM2  (via drill 0.38)
  Top 0.254: THMB.13 33.93,13.52 v33.93,11.68 | v22.89,15.49 22.63,15.75 HAND_MICRO.42
  Route2 0.254: v33.93,11.68 32.64,11.38 27.08,11.38 v22.89,15.49
THAPWM3  (via drill 0.38)
  Top 0.254: THMB1.13 37.82,120.11 v37.82,121.94 | v48.87,118.14 49.13,117.88 HAND_MICRO1.42
  Route2 0.254: v37.82,121.94 39.12,122.25 44.68,122.25 v48.87,118.14
THAPWM4  (via drill 0.38)
  Top 0.254: THMB1.14 37.56,119.28 36.52,119.28 36.14,119.66 36.14,120.14 36.63,120.62 v36.63,122.03 | v49.63,119.28 v49.63,119.27 HAND_MICRO1.41
  Route2 0.254: v36.63,122.03 37.47,122.83 44.93,122.83 48.49,119.28 v49.63,119.28
THAPWM5  (via drill 0.38)
  Top 0.254: THMB2.13 112.67,52.95 v112.67,54.79 | v123.72,50.98 123.98,50.72 HAND_MICRO2.42
  Route2 0.254: v112.67,54.79 113.97,55.09 119.53,55.09 v123.72,50.98
THAPWM6  (via drill 0.38)
  Top 0.254: THMB2.14 112.42,52.12 111.38,52.12 111,52.5 111,52.98 111.48,53.47 v111.48,54.88 | v124.48,52.12 HAND_MICRO2.41
  Route2 0.254: v111.48,54.88 112.32,55.68 119.79,55.68 123.34,52.12 v124.48,52.12
THAPWM7  (via drill 0.38)
  Top 0.254: THMB3.13 108.92,80.53 v108.92,78.69 | v97.87,82.5 97.61,82.76 HAND_MICRO3.42
  Route2 0.254: v108.92,78.69 107.62,78.38 102.06,78.38 v97.87,82.5
THAPWM8  (via drill 0.38)
  Top 0.254: THMB3.14 109.17,81.36 110.21,81.36 110.59,80.97 110.59,80.49 110.11,80.01 v110.11,78.6 | v97.1,81.36 v97.11,81.36 HAND_MICRO3.41
  Route2 0.254: v110.11,78.6 109.27,77.8 101.8,77.8 98.25,81.36 v97.1,81.36
THB1
  Top 0.254: 29.21,15.84 29.36,15.69 THMB.5
  Top 0.635: 29.21,15.84 28.6,16.79 29.21,18.49 30.68,19.23 31.19,20.07 31.8,20.75 34.98,21.74 37.36,22.28 38.73,22.28 39.27,22.73 39.5,24.49 40.34,24.94 40.8,24.87 THUMB_B.2
THB2
  Top 0.381: 32.18,19.61 31.57,18.59 31.55,18.57 THMB.3
  Top 0.635: 32.18,19.61 35.23,20.68 37.97,21.21 39.65,21.21 40.59,22.2 THUMB_B.1
THB3
  Top 0.381: 39.57,114.02 40.18,115.04 40.2,115.06 THMB1.3
  Top 0.635: 39.57,114.02 36.52,112.95 33.78,112.42 32.11,112.42 31.16,111.43 THUMB_B1.1
THB4
  Top 0.254: 42.55,117.79 42.39,117.94 THMB1.5
  Top 0.635: 42.55,117.79 43.16,116.84 42.55,115.14 41.07,114.4 40.56,113.56 39.95,112.88 36.78,111.89 34.39,111.35 33.02,111.35 32.49,110.9 32.26,109.14 31.42,108.69 30.95,108.76 THUMB_B1.2
THB5
  Top 0.381: 114.43,46.86 115.04,47.88 115.06,47.9 THMB2.3
  Top 0.635: 114.43,46.86 111.38,45.8 108.64,45.26 106.96,45.26 106.02,44.27 THUMB_B2.1
THB6
  Top 0.254: 117.4,50.63 117.25,50.78 THMB2.5
  Top 0.635: 117.4,50.63 118.01,49.68 117.4,47.98 115.93,47.24 115.42,46.41 114.81,45.72 111.63,44.73 109.25,44.2 107.87,44.2 107.34,43.74 107.11,41.99 106.27,41.53 105.81,41.6 THUMB_B2.2
THB7
  Top 0.381: 107.16,86.61 106.55,85.6 106.53,85.58 THMB3.3
  Top 0.635: 107.16,86.61 110.21,87.68 112.95,88.21 114.63,88.21 115.57,89.2 THUMB_B3.1
THB8
  Top 0.254: 104.19,82.85 104.34,82.7 THMB3.5
  Top 0.635: 104.19,82.85 103.58,83.8 104.19,85.5 105.66,86.23 106.17,87.07 106.78,87.76 109.96,88.75 112.34,89.28 113.72,89.28 114.25,89.74 114.48,91.49 115.32,91.95 115.78,91.87 THUMB_B3.2
THBENC1
  Top 0.254: HAND_MICRO.51 29.81,20.47 31.17,22.07 36.58,23.44 38.3,26.98 40.16,27.58 40.46,28.5 41.31,28.5 THUMB_B.5
THBENC2
  Top 0.254: HAND_MICRO.50 30.15,19.94 31.39,21.57 36.98,22.96 38.68,26.47 THUMB_B.4
THBENC3
  Top 0.254: HAND_MICRO1.50 41.6,113.69 40.36,112.06 34.77,110.67 33.07,107.16 THUMB_B1.4
THBENC4
  Top 0.254: HAND_MICRO1.51 41.94,113.16 40.59,111.56 35.18,110.19 33.45,106.66 31.6,106.05 31.29,105.13 30.44,105.13 THUMB_B1.5
THBENC5
  Top 0.254: HAND_MICRO2.50 116.46,46.53 115.21,44.91 109.63,43.51 107.92,40.01 THUMB_B2.4
THBENC6
  Top 0.254: HAND_MICRO2.51 116.8,46.01 115.44,44.4 110.03,43.03 108.31,39.5 106.45,38.89 106.15,37.97 105.29,37.97 THUMB_B2.5
THBENC7
  Top 0.254: HAND_MICRO3.50 105.13,86.95 106.38,88.57 111.96,89.97 113.67,93.47 THUMB_B3.4
THBENC8
  Top 0.254: HAND_MICRO3.51 104.79,87.47 106.15,89.08 111.56,90.45 113.28,93.98 115.14,94.59 115.44,95.5 116.3,95.5 THUMB_B3.5
THBISEN  (via drill 0.38)
  Top 0.254: v19.76,26.82 20.13,27.19 HAND_MICRO.12
  Top 0.381: THMB.4 30.67,17.5
  Top 0.635: 30.67,17.5 v30.1,17.68
  Route2 0.254: v30.1,17.68 29.31,16.89 22.55,16.89 21.49,18.41 21.49,24.43 19.76,25.7 v19.76,26.82
  Bottom 0.635: v30.1,17.68 28.83,16.41 R5.2
THBISEN1  (via drill 0.38)
  Top 0.254: v51.99,106.81 51.63,106.44 HAND_MICRO1.12
  Top 0.381: THMB1.4 41.08,116.13
  Top 0.635: 41.08,116.13 v41.66,115.95
  Route2 0.254: v41.66,115.95 42.44,116.74 49.2,116.74 50.27,115.21 50.27,109.19 51.99,107.92 v51.99,106.81
  Bottom 0.635: v41.66,115.95 42.93,117.22 R21.2
THBISEN2  (via drill 0.38)
  Top 0.254: v126.85,39.65 126.48,39.28 HAND_MICRO2.12
  Top 0.381: THMB2.4 115.94,48.97
  Top 0.635: 115.94,48.97 v116.51,48.79
  Route2 0.254: v116.51,48.79 117.3,49.58 124.05,49.58 125.12,48.06 125.12,42.04 126.85,40.77 v126.85,39.65
  Bottom 0.635: v116.51,48.79 117.78,50.06 R37.2
THBISEN3  (via drill 0.38)
  Top 0.254: v94.74,93.83 95.11,94.19 HAND_MICRO3.12
  Top 0.381: THMB3.4 105.65,84.51
  Top 0.635: 105.65,84.51 v105.08,84.68
  Route2 0.254: v105.08,84.68 104.29,83.9 97.54,83.9 96.47,85.42 96.47,91.44 94.74,92.71 v94.74,93.83
  Bottom 0.635: v105.08,84.68 103.81,83.41 R53.2
THBPWM1
  Top 0.254: THMB.7 28.61,14.39 28.37,14.15 28.37,13.64 27.96,13.23 25.81,13.23 24.13,14.91 HAND_MICRO.45
THBPWM2
  Top 0.254: THMB.8 28.64,12.78 25.5,12.78 23.63,14.65 HAND_MICRO.44
THBPWM3
  Top 0.254: THMB1.8 43.12,120.85 46.25,120.85 48.13,118.98 HAND_MICRO1.44
THBPWM4
  Top 0.254: THMB1.7 43.14,119.24 43.38,119.48 43.38,119.99 43.79,120.4 45.95,120.4 47.63,118.72 HAND_MICRO1.45
THBPWM5
  Top 0.254: THMB2.8 117.97,53.7 121.11,53.7 122.98,51.82 HAND_MICRO2.44
THBPWM6
  Top 0.254: THMB2.7 117.99,52.08 118.24,52.32 118.24,52.83 118.64,53.24 120.8,53.24 122.48,51.56 HAND_MICRO2.45
THBPWM7
  Top 0.254: THMB3.8 103.62,79.78 100.48,79.78 98.61,81.66 HAND_MICRO3.44
THBPWM8
  Top 0.254: THMB3.7 103.6,81.4 103.35,81.15 103.35,80.64 102.95,80.24 100.79,80.24 99.11,81.92 HAND_MICRO3.45
USB_D1_N
  Top 0.333: R1.1 13.8,37.13 13.16,37.01 13.16,37.74 13.16,37.75 13.16,38.68 12.73,39.11 D-.P$1 11.36,39.45 10.93,39.45 10.52,39.85 9.07,39.85 8.94,39.98 USB.2
USB_D1_N1
  Top 0.333: R17.1 57.96,96.5 58.6,96.62 58.6,95.89 58.6,95.88 58.6,94.94 59.02,94.52 D-1.P$1 60.4,94.18 60.83,94.18 61.23,93.78 62.69,93.78 62.82,93.65 USB1.2
USB_D1_N2
  Top 0.333: R33.1 132.81,29.34 133.45,29.46 133.45,28.73 133.45,27.79 133.87,27.37 D-2.P$1 135.25,27.02 135.68,27.02 136.09,26.62 137.54,26.62 137.67,26.49 USB2.2
USB_D1_N3
  Top 0.333: R49.1 88.78,104.14 88.14,104.01 88.14,104.75 88.14,105.69 87.72,106.11 D-3.P$1 86.34,106.45 85.91,106.45 85.5,106.86 84.05,106.86 83.92,106.99 USB3.2
USB_D1_P
  Top 0.333: R2.1 12.65,35.65 12.65,37.74 12.24,38.15 D+.P$1 11.28,38.93 11.07,38.94 10.71,38.94 10.31,39.34 9.07,39.34 9.06,39.33 USB.3
USB_D1_P1
  Top 0.333: R18.1 59.11,97.98 59.11,95.89 59.51,95.48 D+1.P$1 60.48,94.7 60.68,94.69 61.04,94.69 61.45,94.29 62.69,94.29 62.7,94.3 USB1.3
USB_D1_P2
  Top 0.333: R34.1 133.96,30.83 133.96,28.73 134.37,28.32 D+2.P$1 135.33,27.54 135.53,27.54 135.89,27.54 136.3,27.13 137.54,27.13 137.55,27.14 USB2.3
USB_D1_P3
  Top 0.333: R50.1 87.63,102.65 87.63,104.75 87.22,105.16 D+3.P$1 86.26,105.93 86.06,105.94 85.69,105.94 85.29,106.35 84.05,106.35 84.04,106.34 USB3.3
USB_D2_N
  Top 0.254: 23.11,28.04 23.13,28.03 HAND_MICRO.6
  Top 0.333: R1.2 13.23,34.3 13.23,32.19 19.43,25.98 22.42,25.98 23.11,26.67 23.11,28.04
USB_D2_N1
  Top 0.254: 48.64,105.59 48.63,105.6 HAND_MICRO1.6
  Top 0.333: R17.2 58.52,99.33 58.52,101.44 52.32,107.64 49.33,107.64 48.64,106.95 48.64,105.59
USB_D2_N2
  Top 0.254: 123.5,38.43 123.48,38.44 HAND_MICRO2.6
  Top 0.333: R33.2 133.37,32.18 133.37,34.29 127.17,40.49 124.19,40.49 123.5,39.8 123.5,38.43
USB_D2_N3
  Top 0.254: 98.09,95.05 98.11,95.04 HAND_MICRO3.6
  Top 0.333: R49.2 88.22,101.3 88.22,99.19 94.42,92.99 97.41,92.99 98.09,93.68 98.09,95.05
USB_D2_P
  Top 0.254: 23.63,28.05 HAND_MICRO.5
  Top 0.333: R2.2 12.18,33.17 12.72,33.17 12.72,31.97 19.22,25.48 22.64,25.48 23.62,26.46 23.62,28.04 23.63,28.05
USB_D2_P1
  Top 0.254: 48.13,105.58 HAND_MICRO1.5
  Top 0.333: R18.2 59.58,100.46 59.03,100.46 59.03,101.66 52.53,108.15 49.12,108.15 48.13,107.17 48.13,105.59 48.13,105.58
USB_D2_P2
  Top 0.254: 122.98,38.42 HAND_MICRO2.5
  Top 0.333: R34.2 134.43,33.3 133.88,33.3 133.88,34.5 127.39,41 123.97,41 122.99,40.01 122.99,38.43 122.98,38.42
USB_D2_P3
  Top 0.254: 98.61,95.05 HAND_MICRO3.5
  Top 0.333: R50.2 87.16,100.18 87.7,100.18 87.7,98.98 94.2,92.48 97.62,92.48 98.6,93.47 98.6,95.05 98.61,95.05
VIN
  Bottom 0.254: 32,38.48 33.95,40.42 U$2.2
  Bottom 1.016: 36.14,44.37 36.68,43.84 36.68,42.85 | 34.72,45.26 34.04,44.58 34.04,42.9 35,43.87 35,44.93
  Bottom 1.27: U$10.B 35.59,42.11 U$2.2
  Bottom 1.905: 32,35.05 32,32.96 33.12,31.84 33.03,31.84 30.14,28.94
  Bottom 2.032: 32,38.48 32,35.05
  pour Bottom (isolate 0.762): 37.06,37.82 37.06,45.97 36.45,46.58 36.45,49.17 35.99,49.63 34.67,49.63 33.25,48.21 31.83,48.21 30.81,47.19 30.81,36.5 30.99,36.32 30.99,33.1 28.85,30.96 28.85,29.06 30.02,27.89 31.52,27.89 33.63,30 33.63,36.83 34.06,37.26 36.5,37.26
VIN1
  Bottom 0.254: 39.75,95.15 37.81,93.2 U$16.2
  Bottom 1.016: 35.61,89.26 35.08,89.79 35.08,90.78 | 37.03,88.37 37.72,89.05 37.72,90.73 36.75,89.76 36.75,88.7
  Bottom 1.27: U$22.B 36.17,91.52 U$16.2
  Bottom 1.905: 39.75,98.58 39.75,100.67 38.63,101.79 38.72,101.79 41.62,104.69
  Bottom 2.032: 39.75,95.15 39.75,98.58
  pour Bottom (isolate 0.762): 34.7,95.81 34.7,87.66 35.31,87.05 35.31,84.45 35.76,84 37.08,84 38.51,85.42 39.93,85.42 40.94,86.44 40.94,97.13 40.77,97.31 40.77,100.53 42.9,102.67 42.9,104.57 41.73,105.74 40.23,105.74 38.13,103.63 38.13,96.8 37.69,96.37 35.26,96.37
VIN2
  Bottom 0.254: 114.61,27.99 112.66,26.05 U$28.2
  Bottom 1.016: 110.47,22.1 109.93,22.63 109.93,23.62 | 111.89,21.21 112.57,21.89 112.57,23.57 111.61,22.61 111.61,21.54
  Bottom 1.27: U$34.B 111.02,24.36 U$28.2
  Bottom 1.905: 114.61,31.42 114.61,33.52 113.49,34.63 113.58,34.63 116.47,37.53
  Bottom 2.032: 114.61,27.99 114.61,31.42
  pour Bottom (isolate 0.762): 109.55,28.65 109.55,20.5 110.16,19.89 110.16,17.3 110.62,16.84 111.94,16.84 113.36,18.26 114.78,18.26 115.8,19.28 115.8,29.97 115.62,30.15 115.62,33.38 117.75,35.51 117.75,37.41 116.59,38.58 115.09,38.58 112.98,36.47 112.98,29.64 112.55,29.21 110.11,29.21
VIN3
  Bottom 0.254: 106.98,105.49 108.93,107.43 U$40.2
  Bottom 1.016: 111.12,111.38 111.66,110.85 111.66,109.86 | 109.7,112.27 109.02,111.58 109.02,109.91 109.98,110.87 109.98,111.94
  Bottom 1.27: U$46.B 110.57,109.12 U$40.2
  Bottom 1.905: 106.98,102.06 106.98,99.96 108.1,98.84 108.01,98.84 105.12,95.95
  Bottom 2.032: 106.98,105.49 106.98,102.06
  pour Bottom (isolate 0.762): 112.04,104.83 112.04,112.98 111.43,113.59 111.43,116.18 110.97,116.64 109.65,116.64 108.23,115.21 106.81,115.21 105.79,114.2 105.79,103.5 105.97,103.33 105.97,100.1 103.84,97.97 103.84,96.06 105,94.89 106.5,94.89 108.61,97 108.61,103.84 109.04,104.27 111.48,104.27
